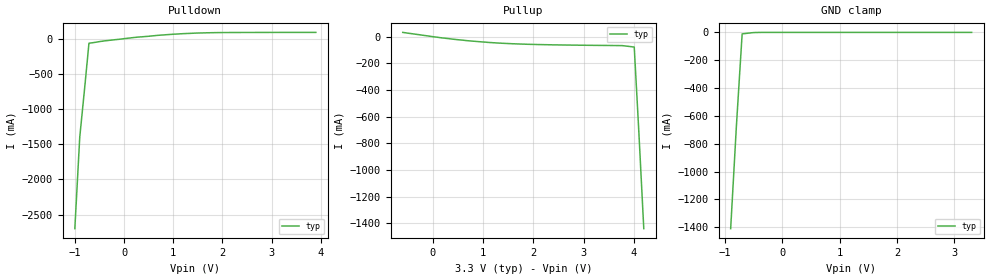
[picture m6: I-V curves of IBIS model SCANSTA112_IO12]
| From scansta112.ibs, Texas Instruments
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|   3-State Input/Output 12mA MODEL
[Model]   SCANSTA112_IO12
Model_type   I/O
Vinh = 2.1
Vinl = 0.8
Vmeas =   1.25
| Variable   typ   min   max
C_comp   5.00pF   NA   NA
|   typ   min   max
[Temperature Range]   25.0   NA   NA
[Voltage range]   3.3V   NA   NA
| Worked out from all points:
|   slope of the pulldown table from 0 to 0.495 V, typ, clamps not added: 14.7 ohm
|   slope of the pullup table from 0 to 0.495 V, typ, clamps not added: 21.9 ohm
|   GND clamp passes 1 mA (typ) near -0.47 V on its own axis
[Pulldown]
| Voltage   I(typ)   I(min)   I(max)
-1V       -2.7A      NA         NA
-900mV    -1.4A      NA         NA
-800mV    -700mA     NA         NA
-713mV    -65mA      NA         NA
200mV     16mA       NA         NA
1.2V      71mA       NA         NA
2V        87mA       NA         NA
3.9V      89mA       NA         NA
[Pullup]
| Voltage   I(typ)   I(min)   I(max)
-600mV    32.15mA    NA         NA
400mV     -18.68mA   NA         NA
1.3V      -47.73mA   NA         NA
2.1V      -59mA      NA         NA
3.765V    -66.99mA   NA         NA
4.01V     -77.88mA   NA         NA
4.1V      -702mA     NA         NA
4.2V      -1.44A     NA         NA
[GND_clamp]
| Outputs in Tri-state
| Voltage   I(typ)   I(min)   I(max)
-900mV    -1.41A     NA         NA
-800mV    -672mA     NA         NA
-700mV    -10.6mA    NA         NA
-400mV    -203uA     NA         NA
3.3V      492pA      NA         NA
[POWER_clamp]
| Voltage   I(typ)   I(min)   I(max)
-3.3V     0A         NA         NA
3.3V      0A         NA         NA
[Ramp]
|   typ   min   max
dV/dt_r   1.889/1.60n   NA   NA
dV/dt_f   1.889/0.90n   NA   NA
|[Cload] = 30pF
R_load = 500ohms
